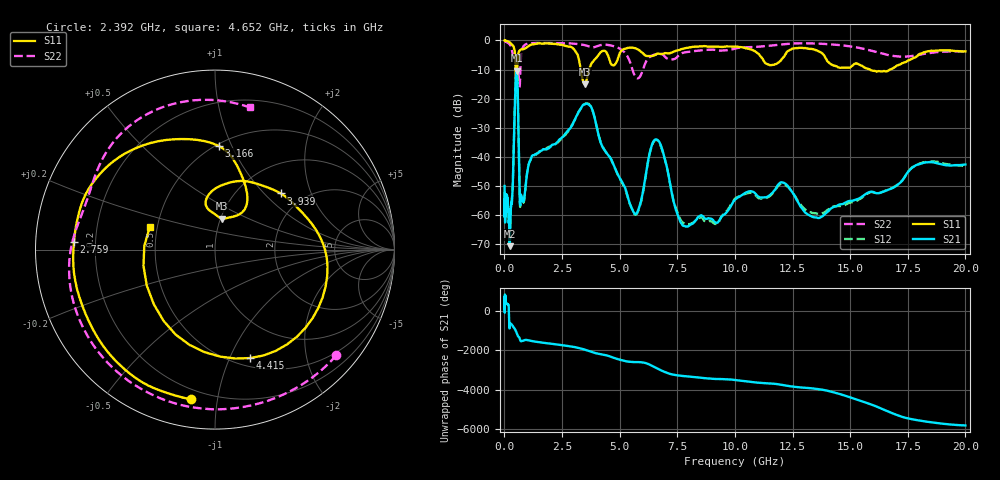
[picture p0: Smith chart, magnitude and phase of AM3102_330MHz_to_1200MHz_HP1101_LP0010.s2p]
! Date/Time: Tue, Sep 11, 2018 5:22 PM
! Network Analyzer: Agilent Technologies E8362B Rev: A.07.50.63
! Sweep from 0.010 to 20.000 GHz, 1601 Points, Sweep Type: LOG
! Power Supply: 4.949 V, 0.001 A
# Hz S DB R 50
!freq MagS11 AngS11 MagS21 AngS21 MagS12 AngS12 MagS22 AngS22
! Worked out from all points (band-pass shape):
!   1601 points, 10 MHz to 20 GHz, reference 50 ohm
!   highest |S21| = -10.40 dB at 528.1 MHz (marker M1); lowest = -70.6 dB at 233.3 MHz (marker M2)
!   |S21| within 3 dB of the highest: 492.1 MHz to 561.6 MHz (69.47 MHz wide, 13.2 % of centre)
!   lowest |S11| = -15.1 dB at 3.482 GHz (marker M3), VSWR 1.43, Z = 50.7 + j18 ohm
!   |S11| at or under -10 dB: 486.5 MHz to 556.2 MHz (69.69 MHz wide, 13.4 % of centre); 3.314 GHz to 3.676 GHz (361.7 MHz wide, 10.4 % of centre); 15.86 GHz to 16.74 GHz (873.7 MHz wide, 5.36 % of centre)
!   |S22| runs from -16.1 to -0.1 dB; largest |S21 - S12| = 0.0044
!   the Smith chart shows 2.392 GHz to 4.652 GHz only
!   S11 on the Smith chart (normalised r, x): 2.392 GHz: 0.14, -0.84; 2.759 GHz: 0.12, +0.03; 3.166 GHz: 0.52, +0.89; 3.939 GHz: 1.54, +1.25; 4.415 GHz: 0.59, -1.19; 4.652 GHz: 0.45, +0.13
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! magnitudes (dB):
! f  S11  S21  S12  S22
! 10 MHz  0.0  -50.0  -58.5  -0.1
! 35.55 MHz  -0.1  -59.6  -58.3  -0.3
! 126.4 MHz  -0.2  -54.9  -56.1  -0.7
! 233.3 MHz  -0.7  -70.6  -69.6  -1.4
! 357.7 MHz  -1.7  -51.0  -51.4  -4.7
! 447.2 MHz  -3.5  -24.5  -24.5  -4.2
! 528.1 MHz  -13.5  -10.4  -10.4  -11.0
! 682.6 MHz  -3.3  -56.5  -57.1  -13.0
! 1.59 GHz  -1.0  -37.9  -37.8  -0.9
! 2.392 GHz  -1.5  -33.9  -34.4  -0.9
! 2.759 GHz  -2.1  -31.0  -31.3  -1.0
! 3.166 GHz  -4.8  -25.4  -25.4  -1.2
! 3.482 GHz  -15.1  -22.0  -21.8  -1.6
! 3.939 GHz  -6.3  -27.3  -27.3  -2.2
! 4.415 GHz  -3.9  -38.5  -38.4  -1.5
! 4.652 GHz  -8.3  -41.1  -41.2  -1.8
! 5.652 GHz  -2.6  -59.5  -59.7  -12.1
! 6.58 GHz  -4.8  -34.0  -34.2  -4.8
! 7.92 GHz  -2.5  -63.9  -63.1  -4.0
! 12.03 GHz  -6.5  -48.6  -49.1  -1.4
! 13.61 GHz  -3.7  -61.0  -59.4  -1.1
! 20 GHz  -3.8  -42.6  -43.1  -3.8
